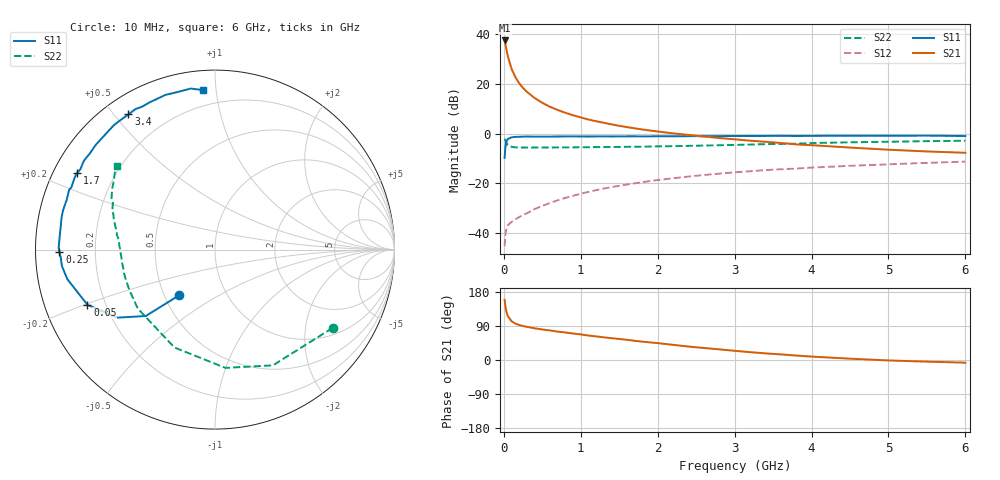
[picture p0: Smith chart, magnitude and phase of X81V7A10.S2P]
! SIEMENS Small Signal Semiconductors
! BFP136W
! Si NPN RF Bipolar Junction Transistor in SOT343
! VCE = 1.75 V  IC = 100 mA
! Common Emitter S-Parameters:  September  1994
# GHz  S  MA  R  50
!  f  S11  S21  S12  S22
! GHz  MAG  ANG  MAG  ANG  MAG  ANG  MAG  ANG
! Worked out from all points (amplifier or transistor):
!   40 points, 10 MHz to 6 GHz, reference 50 ohm
!   highest |S21| = 37.5 dB at 10 MHz (marker M1)
!   |S21| within 3 dB of that: start of sweep to 29.49 MHz
!   unconditionally stable (mu >= 1): 459.2 MHz to 2.916 GHz
!   at 200 MHz: K = 0.72, MSG = 26.9 dB, |S12| = -33.6 dB
!   at 1.5 GHz: K = 1.11, MAG = 10.0 dB, |S12| = -21.0 dB
!   at 6 GHz: K = 0.99, MSG = 1.8 dB, |S12| = -11.3 dB
!   S11 on the Smith chart (normalised r, x): 10 MHz: 0.60, -0.34; 50 MHz: 0.13, -0.20; 250 MHz: 0.07, -0.01; 1.7 GHz: 0.07, +0.26; 3.4 GHz: 0.07, +0.55; 6 GHz: 0.11, +0.92
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0.01  0.3235 -128.1  74.86 159.0  0.0054 68.1  0.787 -33.7
0.02  0.5346 -136.2  63.37 141.8  0.0092 54.5  0.7211 -63.4
0.03  0.6627 -145.1  52.48 130.0  0.0115 46.8  0.6616 -84.9
0.05  0.7743 -156.6  36.88 116.2  0.0142 37.4  0.5902 -112.6
0.1  0.8392 -168.7  20.15 102.4  0.0166 36.2  0.5411 -142.7
0.15  0.8582 -174.0  13.66 96.1  0.0187 39.7  0.5274 -154.8
0.2  0.8597 -176.7  10.25 92.4  0.0209 42.5  0.5241 -161.2
0.25  0.8673 -179.2  8.265 89.6  0.0229 46.8  0.5236 -165.3
0.3  0.8713 179.4  6.907 87.5  0.0248 48.9  0.5217 -168.0
0.4  0.8685 175.9  5.196 83.7  0.0302 53.5  0.5228 -171.7
0.5  0.8685 173.5  4.147 80.5  0.0349 57.0  0.5228 -174.3
0.6  0.8688 171.5  3.458 78.0  0.0401 59.2  0.5241 -176.0
0.7  0.872 169.1  2.982 74.9  0.0453 60.6  0.5254 -177.3
0.9  0.8742 165.6  2.336 69.9  0.0558 61.8  0.5273 -179.7
1.1  0.8716 161.4  1.914 64.5  0.067 62.1  0.531 178.6
1.7  0.8797 151.0  1.275 50.6  0.0993 59.6  0.5424 173.7
2.2  0.8792 142.6  1.01 40.0  0.1258 55.6  0.5563 169.8
3.2  0.8933 125.7  0.718 20.7  0.1741 45.8  0.5991 160.9
3.4  0.8948 122.6  0.682 17.5  0.1839 43.6  0.6121 159.1
4.5  0.9052 107.7  0.522 3.5  0.2239 33.1  0.6661 149.3
5.5  0.9076 98.6  0.436 -4.3  0.2568 25.1  0.7028 142.6
6  0.8911 94.3  0.41 -7.1  0.2726 20.7  0.7164 139.6
